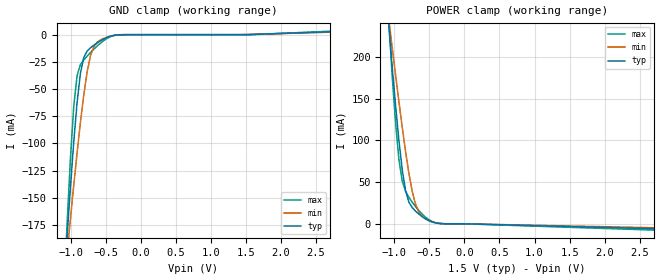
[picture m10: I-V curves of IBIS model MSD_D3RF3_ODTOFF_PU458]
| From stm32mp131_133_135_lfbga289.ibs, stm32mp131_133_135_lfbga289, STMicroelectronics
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[Model] MSD_D3RF3_ODTOFF_PU458
Model_type   Input
C_comp 2.387pF   2.305pF   2.510pF
Vinh = 925.000mV
Vinl = 575.000mV
[Temperature Range]   25.000   125.000   -40.000
[Voltage Range]   1.500V   1.425V   1.575V
[GND Clamp Reference]   0.00V   0.00V   0.00V
[POWER Clamp Reference]   1.500V   1.425V   1.575V
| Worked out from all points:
|   GND clamp passes 1 mA (typ) near -0.40 V on its own axis
|   POWER clamp passes 1 mA (typ) near -0.41 V on its own axis
[GND Clamp]
-1.48V    -635.6mA   -502.6mA   -842.5mA
-1.098V   -233.7mA   -234.3mA   -242.8mA
-1.05V    -186.3mA   -201.7mA   -175.2mA
-1.002V   -140.9mA   -169.8mA   -114.4mA
-954.6mV  -98.84mA   -138.7mA   -66.04mA
-906.8mV  -62.47mA   -108.8mA   -37.58mA
-859.1mV  -35.55mA   -80.71mA   -27.52mA
-811.4mV  -20.94mA   -55.39mA   -23.21mA
-715.9mV  -12.03mA   -19.45mA   -16.48mA
-572.7mV  -5.676mA   -4.812mA   -7.763mA
-286.4mV  -68.41uA   -114.8uA   -53.22uA
2.959V    3.23mA     2.75mA     3.905mA
[Power Clamp]
-1.459V   642.5mA    516.9mA    840.2mA
-1.077V   236.3mA    244.5mA    242mA
-1.03V    188.1mA    211.3mA    177.5mA
-981.8mV  142.1mA    178.6mA    120.9mA
-934.1mV  100mA      146.6mA    77.12mA
-886.4mV  64.64mA    115.6mA    51.01mA
-838.6mV  39.34mA    86.4mA     38.95mA
-743.2mV  19.32mA    38.46mA    25.85mA
-647.7mV  11.51mA    13.71mA    15.66mA
-552.3mV  5.8mA      5.717mA    7.762mA
-313.6mV  106.5uA    244.9uA    120.3uA
2.98V     -6.503mA   -5.233mA   -8.321mA
